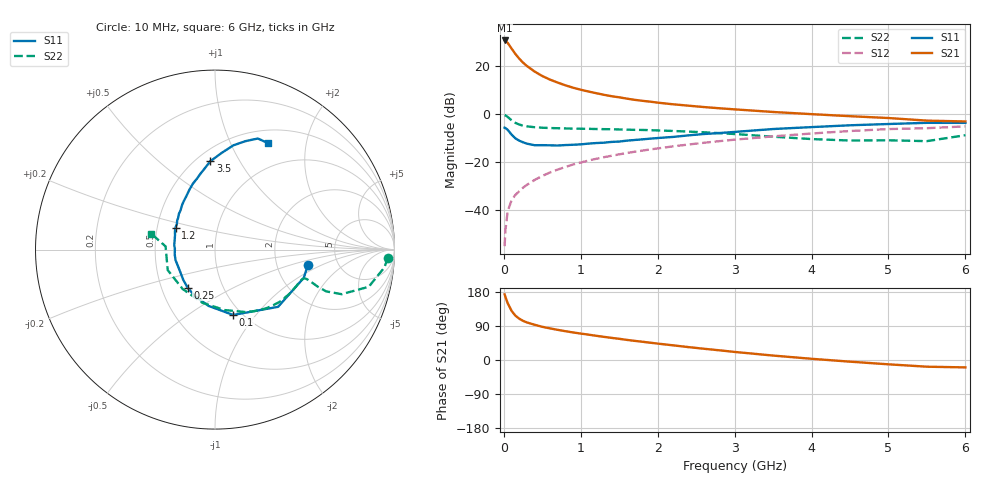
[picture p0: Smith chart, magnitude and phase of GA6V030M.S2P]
! Infineon Technologies  Discrete & RF Semiconductors
! BF775
! Si NPN RF Bipolar Junction Transistor in SOT23
! VCE = 6 V  IC = 30 mA
! Common Emitter S-Parameters:  May  1996
# GHz  S  MA  R  50
!  f  S11  S21  S12  S22
! GHz  MAG  ANG  MAG  ANG  MAG  ANG  MAG  ANG
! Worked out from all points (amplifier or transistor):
!   36 points, 10 MHz to 6 GHz, reference 50 ohm
!   highest |S21| = 30.7 dB at 10 MHz (marker M1)
!   |S21| within 3 dB of that: start of sweep to 92.48 MHz
!   unconditionally stable (mu >= 1): 300.6 MHz to 2.754 GHz
!   at 250 MHz: K = 0.94, MSG = 26.0 dB, |S12| = -30.5 dB
!   at 1.4 GHz: K = 1.12, MAG = 10.3 dB, |S12| = -17.3 dB
!   at 6 GHz: K = 0.94, MSG = 1.0 dB, |S12| = -5.0 dB
!   S11 on the Smith chart (normalised r, x): 10 MHz: 3.03, -0.69; 100 MHz: 0.91, -0.77; 250 MHz: 0.68, -0.31; 1.2 GHz: 0.62, +0.16; 3.5 GHz: 0.58, +0.76; 6 GHz: 0.66, +1.40
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0.01  0.5249 -9.1  34.34 173.2  0.0018 94.2  0.9643 -2.7
0.02  0.5191 -17.6  33.68 166.8  0.0038 83.1  0.9492 -6.0
0.05  0.4746 -42.2  30.55 149.9  0.0096 74.8  0.8812 -13.6
0.1  0.3778 -74.5  23.35 129.8  0.0161 67.6  0.748 -19.4
0.15  0.3158 -96.5  18.02 117.0  0.021 66.9  0.662 -20.6
0.2  0.2819 -113.4  14.38 109.1  0.0249 68.0  0.6113 -19.9
0.25  0.261 -125.8  11.86 103.3  0.0297 68.8  0.5794 -19.0
0.3  0.2447 -136.1  10.11 99.1  0.034 70.2  0.5603 -18.5
0.4  0.2269 -152.5  7.745 93.0  0.043 71.4  0.5375 -17.8
0.5  0.2276 -165.1  6.238 87.6  0.0521 72.8  0.5244 -17.8
0.6  0.226 -173.2  5.266 83.4  0.0615 72.9  0.5175 -18.3
0.7  0.2236 178.3  4.561 79.6  0.0707 73.1  0.5121 -19.0
0.8  0.2286 173.7  4.005 76.0  0.08 72.6  0.507 -20.1
0.9  0.2319 165.3  3.571 72.7  0.0901 72.3  0.5023 -21.2
1.1  0.2451 155.6  2.972 66.9  0.1088 71.3  0.4972 -24.1
1.2  0.2519 150.8  2.748 63.9  0.1184 70.6  0.4934 -25.4
1.7  0.2914 131.1  1.997 50.5  0.166 66.4  0.4738 -33.8
2.2  0.3378 118.2  1.613 38.7  0.2149 61.6  0.4491 -43.6
3.5  0.493 93.0  1.116 11.7  0.3468 46.4  0.3415 -80.7
4.5  0.5899 80.0  0.912 -4.4  0.4482 32.8  0.284 -129.4
5.5  0.6634 68.9  0.737 -17.7  0.5129 16.4  0.2759 176.3
6  0.6625 63.5  0.709 -19.5  0.5599 11.8  0.3667 165.9
